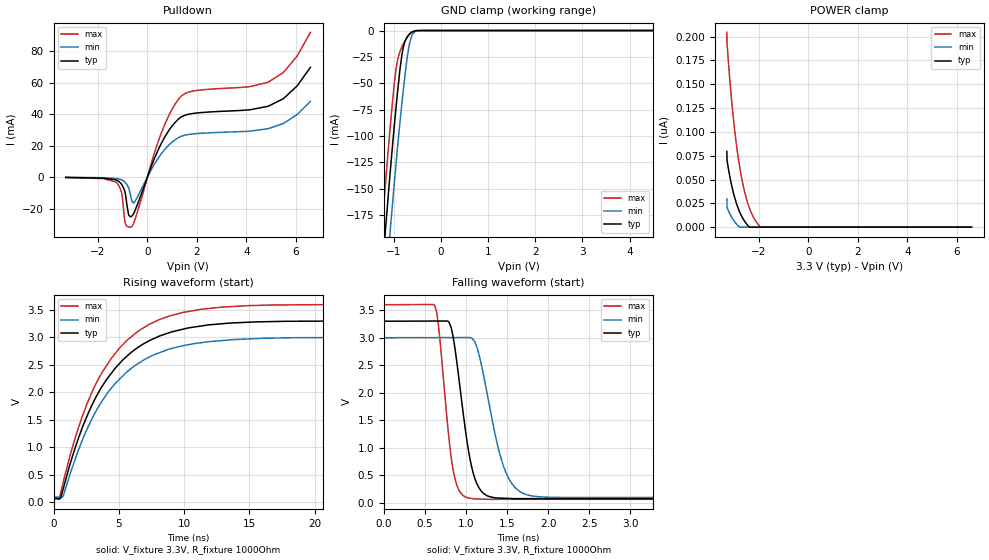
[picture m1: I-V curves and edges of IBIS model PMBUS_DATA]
| Texas Instruments Incorporated
| Digital Controller for Isolated Power
| Part#   Voltage Range   #pins
| UCD3138128APFC   3.0V - 3.6V   80
[IBIS ver]   4.0
[File name]   ucd3138128.ibs
[File Rev]   1.0
[Date]   11/16/2017
[Source]   Texas Instruments Incorporated.
   Analog_eLab, HPA
   12500 TI Blvd
   Dallas, TX _75243
[Notes]   Revision History
   Rev 11/16/2017
   - Initial version of the model
[Disclaimer] This model is designed as an aid for customers of Texas Instruments.
 TI and its licensors and suppliers make no warranties, either expressed
 or implied, with respect to this  model, including the warranties of
 merchantability or fitness for a particular purpose.
 The model is provided solely on an "as is" basis. The entire risk as to
 its quality and performance is with the customer.
[Copyright] (C)Copyright 2017 Texas Instruments Incorporated.
   All rights reserved.
|   Component UCD3138128APFC
[Component]   UCD3138128APFC
[Manufacturer]  Texas Instruments Incorporated
[Package]  |  80 pin  PFC
|   typ   min   max
R_pkg   0.067   0.027   0.083
L_pkg   0.937nH   0.593nH   1.143nH
C_pkg   0.144pF   0.126pF   0.200pF
[Pin] signal_name   model_name   R_pin   L_pin   C_pin
1   AD13   TERM   NA   NA   NA
2   AD12   TERM   NA   NA   NA
3   AD10   TERM   NA   NA   NA
4   AD07   TERM   NA   NA   NA
5   AD06   TERM   NA   NA   NA
6   AD04   TERM   NA   NA   NA
7   AD03   TERM   NA   NA   NA
8   V33DIO   POWER   NA   NA   NA
9   DVSS   GND   NA   NA   NA
10   nRESET   TERM   NA   NA   NA
11   PWM-2   TERM   NA   NA   NA
12   PWM-3   TERM   NA   NA   NA
13   TCAP-1   TERM   NA   NA   NA
14   Ext_Trig   TERM   NA   NA   NA
15   PMBus_Clk   PMBUS_DATA   NA   NA   NA
16   PMBus_Data   PMBUS_DATA   NA   NA   NA
17   PMBus_Alert   TERM   NA   NA   NA
18   PMBus_Cntrl   TERM   NA   NA   NA
19   I2C_Clk   TERM   NA   NA   NA
20   I2C_Data   TERM   NA   NA   NA
21   DVSS   GND   NA   NA   NA
22   DPWM-0A   TERM   NA   NA   NA
23   DPWM-0B   TERM   NA   NA   NA
24   DPWM-1A   TERM   NA   NA   NA
25   DPWM-1B   TERM   NA   NA   NA
26   DPWM-2A   TERM   NA   NA   NA
27   DPWM-2B   TERM   NA   NA   NA
28   DPWM-3A   TERM   NA   NA   NA
29   DPWM-3B   TERM   NA   NA   NA
30   GPIO-A   TERM   NA   NA   NA
31   GPIO-B   TERM   NA   NA   NA
32   GPIO-C   TERM   NA   NA   NA
33   GPIO-D   TERM   NA   NA   NA
34   SYNC   TERM   NA   NA   NA
35   SCI_TX-0   TERM   NA   NA   NA
36   SCI_RX-0   TERM   NA   NA   NA
37   SCI_TX-1   TERM   NA   NA   NA
38   SCI_RX-1   TERM   NA   NA   NA
39   PWM-0   TERM   NA   NA   NA
40   PWM-1   TERM   NA   NA   NA
41   DVSS   GND   NA   NA   NA
42   Ext_Int   TERM   NA   NA   NA
43   Fault-0   TERM   NA   NA   NA
44   Fault-1   TERM   NA   NA   NA
45   TCK   TERM   NA   NA   NA
46   TDO   TERM   NA   NA   NA
47   TDI   TERM   NA   NA   NA
48   TMS   TERM   NA   NA   NA
49   TCAP-0   TERM   NA   NA   NA
50   SPI_CS   TERM   NA   NA   NA
51   SPI_CLK   TERM   NA   NA   NA
52   SPI_MOSI   TERM   NA   NA   NA
53   SPI_MISO   TERM   NA   NA   NA
54   Fault-2   TERM   NA   NA   NA
55   Fault-3   TERM   NA   NA   NA
56   DVSS   GND   NA   NA   NA
57   V33DIO   POWER   NA   NA   NA
58   DVDD   POWER   NA   NA   NA
59   V33D   POWER   NA   NA   NA
60   DVSS-A   GND   NA   NA   NA
61   XTAL_Out   TERM   NA   NA   NA
62   XTAL_In   TERM   NA   NA   NA
63   AVSS   GND   NA   NA   NA
64   EAp0   TERM   NA   NA   NA
65   EAn0   TERM   NA   NA   NA
66   EAp1   TERM   NA   NA   NA
67   EAn1   TERM   NA   NA   NA
68   EAp2   TERM   NA   NA   NA
69   EAn2   TERM   NA   NA   NA
70   AVSS   GND   NA   NA   NA
71   V33A   POWER   NA   NA   NA
72   AD00   TERM   NA   NA   NA
73   AD01   TERM   NA   NA   NA
74   AD02   TERM   NA   NA   NA
75   AD05   TERM   NA   NA   NA
76   AD14   TERM   NA   NA   NA
77   AD08   TERM   NA   NA   NA
78   AD09   TERM   NA   NA   NA
79   AD11   TERM   NA   NA   NA
80   AVSS   GND   NA   NA   NA
[Model] TERM
Model_type Terminator
C_comp   0  0  0
| variable   typ   min   max
[Voltage Range]   3.30000V  3.00000V  3.60000V
[POWER Clamp Reference]  3.30000V  3.00000V  3.60000V
[GND Clamp Reference]   0.00000V  0.00000V  0.00000V
[Temperature Range]   27   110   -40
| Models and submodels in the file (2): TERM (Terminator), PMBUS_DATA (I/O_open_drain)
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|   PMBUS_DATA 3.3V Model
[Model]   PMBUS_DATA
Model_type   I/O_open_drain
Polarity   Non-Inverting
Enable   Active-Low
Vinl = 1.1
Vinh = 2.1
Vmeas = 1.65
Vref = 3.3
Cref = 1pF
Rref = 1000
|   typ   min   max
C_comp   1pF   1pF   1pF
[Voltage Range]   3.3   3   3.6
[Temperature Range]   27   110   -40
[Pullup Reference]   3.3   3   3.6
[Pulldown Reference]   -0   -0   -0
[Power Clamp Reference]   3.3   3   3.6
[GND Clamp Reference]   -0   -0   -0
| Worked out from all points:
|   slope of the pulldown table from 0 to 0.495 V, typ, clamps not added: 25.6 ohm
|   GND clamp passes 1 mA (typ) near -0.59 V on its own axis
|   falling waveform, V_fixture 3.3V, R_fixture 1000Ohm: 20-80 % time 180ps typ, 255ps min, 138ps max; typ from 3.3 V to 0.072 V
|   rising waveform, V_fixture 3.3V, R_fixture 1000Ohm: 20-80 % time 4.3ns typ, 4.36ns min, 4.22ns max; typ from 0.072 V to 3.3 V
[Pulldown]
|   Voltage   I(typ)   I(min)   I(max)
-3.3V     -161.6uA   -95.67uA   -239.5uA
-1.28V    -1.688mA   -780.9uA   -3.006mA
-1.043V   -4.549mA   -1.684mA   -9.829mA
-884.4mV  -11.01mA   -3.591mA   -29.97mA
-765.6mV  -23.48mA   -6.398mA   -31.6mA
-656.7mV  -25.05mA   -13.37mA   -31.63mA
-518.1mV  -21.9mA    -15.78mA   -27.67mA
561mV     21.41mA    14.86mA    28.02mA
1.323V    37.81mA    25.68mA    50.76mA
4.887V    45.12mA    30.85mA    60.42mA
5.511V    50.12mA    34.31mA    66.83mA
6.59V     69.87mA    48.23mA    92.11mA
[GND Clamp]
|   Voltage   I(typ)   I(min)   I(max)
-3.3V     -1.479A    -1.52A     -1.447A
-1.261V   -239.9mA   -295.8mA   -196mA
-1.191V   -200.6mA   -256.8mA   -156.7mA
-1.073V   -135.8mA   -191.5mA   -92.9mA
-983.4mV  -90.47mA   -144.9mA   -50.45mA
-943.8mV  -71.69mA   -125.1mA   -35.8mA
-825mV    -24.03mA   -70.22mA   -15.79mA
-765.6mV  -11.57mA   -45.93mA   -10.55mA
-696.3mV  -5.224mA   -21.46mA   -5.541mA
-646.8mV  -2.766mA   -9.894mA   -2.862mA
-587.4mV  -983.3uA   -3.003mA   -890.3uA
6.59V     0A         0A         0A
[POWER Clamp]
|   Voltage   I(typ)   I(min)   I(max)
-3.3V     79.58nA    29.7nA     204.5nA
-3.29V    69.72nA    20.6nA     192.8nA
-3.251V   63.41nA    18.06nA    178.4nA
-3.161V   50.81nA    13.07nA    149nA
-3.072V   40.14nA    8.944nA    123.6nA
-2.924V   26nA       3.641nA    88.97nA
-2.756V   14.39nA    0A         59.34nA
-2.587V   6.336nA    0A         37.76nA
-2.369V   0A         0A         18.8nA
-2.211V   0A         0A         9.654nA
-1.944V   0A         0A         189.8pA
6.59V     0A         0A         0A
[Ramp]
R_load = 1000
|   typ   min   max
dV/dt_r   1.93678/4.28869e-09   1.74422/4.35666e-09   2.12337/4.22655e-09
dV/dt_f   1.93678/1.79918e-10   1.74422/2.54903e-10   2.12337/1.37977e-10
[Falling Waveform]
V_fixture = 3.3V
V_fixture_min = 3V
V_fixture_max = 3.6V
R_fixture = 1000Ohm
C_fixture = 0F
|   Time   V(typ)   V(min)   V(max)
0s        3.3V       3V         3.6V
617.7ps   3.303V     3.002V     3.582V
667.7ps   3.304V     3.002V     3.152V
791.7ps   3.281V     3.003V     1.153V
894.3ps   2.463V     3.003V     288.1mV
1.064ns   669.3mV    2.995V     75.29mV
1.259ns   123.6mV    1.953V     61.81mV
1.553ns   75.2mV     355.7mV    61.81mV
2.172ns   73.59mV    94.98mV    61.81mV
200ns     72.03mV    92.96mV    61.06mV
[Rising Waveform]
V_fixture = 3.3V
V_fixture_min = 3V
V_fixture_max = 3.6V
R_fixture = 1000Ohm
C_fixture = 0F
|   Time   V(typ)   V(min)   V(max)
0s        72.03mV    92.96mV    61.06mV
429.4ps   64.2mV     90.24mV    51.25mV
728.9ps   232.4mV    102.5mV    348mV
1.72ns    1.033V     825.7mV    1.218V
2.956ns   1.773V     1.524V     2.01V
4.042ns   2.227V     1.955V     2.481V
5.071ns   2.53V      2.245V     2.811V
8.102ns   3.025V     2.721V     3.326V
12.92ns   3.251V     2.945V     3.554V
200ns     3.3V       3V         3.6V
